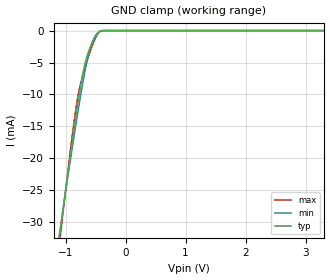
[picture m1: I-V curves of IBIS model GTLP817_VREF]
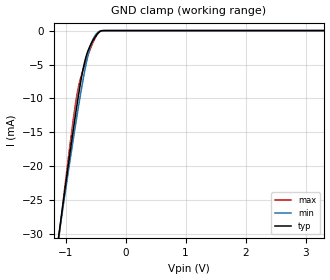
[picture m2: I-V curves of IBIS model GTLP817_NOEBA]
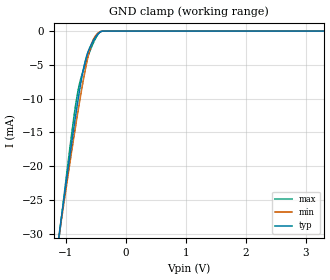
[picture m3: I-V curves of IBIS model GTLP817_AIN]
| TEXAS INSTRUMENTS INCORPORATED
| Standard Linear and Logic Group
| IBIS Model of SN74GTLP817
| GTLP-TO-LVTTL 1-TO-6 FANOUT DRIVER
| This file contains package information for the following:
|  TSSOP 24-pin (PW) package as [Component] GTLP817_PW
|  SOIC 24-pin (DW) package as [Component] GTLP817_DW
|  TVSOP 24-pin (DGV) package as [Component] GTLP817_DGV
| This device can be powered at the following Vccs:
|  3.3 volt Vcc
| This file provides unique models under the [Model Selector] for each Vcc.
| For operation at a specific Vcc, select the appropriate model after each
| [Model Selector] keyword.
[IBIS Ver]   3.2
[Comment char]  |_char
[File Name]   sn74gtlp817.ibs
[File Rev]   1.1 | c_die
[Date]   February 12, 2001
[Source]   Data created from TI-SPICE simulations at TI-SLL.
[Notes]   The following is an IBIS list for the GTLP817.
   Please contact sllibis@ti.com with questions and
   comments concerning SLL IBIS models.
   B_port output is simulated in Slow Mode(ERC=VCC)
   WARNING WHEN IBISCHK3.2.6 is Run
   -Pulldown Maximum data is non-monotonic
   -Pullup Maximum data is non-monotonic
   -Pullup Typical data is non-monotonic
   -Pullup Minimum data is non-monotonic
   -[Model] GTLP817_BOUT has no description of the
   buffer's high state DC drive characteristics
   (no [Pullup] table).This warning can be silenced
   by changing the Model_type or by adding a
   Pullup] table.
[Disclaimer] Property of Texas Instruments Incorporated.  Unauthorized
   reproduction and/or distribution is strictly prohibited.
   This product is protected under copyright law.
   Created  2001, (C) Copyright  2001, Texas Instruments
   Incorporated, All Rights Reserved
   UNLESS THERE IS A SIGNED, WRITTEN AGREEMENT TO THE
   CONTRARY, TEXAS INSTRUMENTS (TI) IS PROVIDING THE IBIS
   MODELS  AND WITHOUT ANY WARRANTY, EXPRESSED OR
   IMPLIED.  TI assumes no liability for:
   1) the accuracy of the IBIS models provided to your
   company;
   2) the proper functioning of these IBIS Models in your
   design or for any resulting applications; or
   3) infringement of patents, copyrights or intellectual
   property rights resulting from your use of these IBIS
   models.
   TI provides IBIS Models as a service to our customers.
   You and your company shall not distribute, sell or give
   these models to anyone else without prior written
   permission from TI.
   TI reserves the right to make changes to our products or
   to discontinue any semiconductor product or service
   without notice, and advises our customers to obtain the
   latest version of relevant information to verify, before
   placing orders, that the information being relied on is
   current.
   Please be aware that your receipt and use of the IBIS
   information provided shall serve as acceptance of these
   terms and conditions.  If you do not accept these terms,
   you should return or destroy the IBIS models and any
   other accompanying information immediately.
| Component GTLP817_PW 24-pin TSSOP
[Component]   GTLP817_PW
[Manufacturer]   Texas Instruments, Inc.
[Package]
|   typ   min   max
R_pkg   3.900e-02   3.000e-02   4.600e-02
L_pkg   2.685e-09   2.367e-09   3.177e-09
C_pkg   3.200e-13   2.520e-13   4.340e-13
[Pin]   signal_name   model_name   R_pin   L_pin   C_pin
1   AI   GTLP817_AIN   3.700e-02   3.153e-09   4.340e-13
2   AO1   GTLP817_AOUT   3.400e-02   2.629e-09   3.410e-13
3   GNDT   GND   3.200e-02   2.860e-09   3.470e-13
4   AO2   GTLP817_AOUT   4.200e-02   2.741e-09   2.900e-13
5   VCC   POWER   4.600e-02   2.600e-09   2.620e-13
6   AO3   GTLP817_AOUT   4.300e-02   2.414e-09   2.660e-13
7   GNDT   GND   4.200e-02   2.367e-09   2.620e-13
8   AO4   GTLP817_AOUT   4.400e-02   2.461e-09   2.520e-13
9   VCC   POWER   4.200e-02   2.543e-09   2.740e-13
10   AO5   GTLP817_AOUT   3.000e-02   2.616e-09   3.320e-13
11   GNDT   GND   3.700e-02   2.670e-09   3.460e-13
12   AO6   GTLP817_AOUT   3.900e-02   3.177e-09   4.330e-13
13   GNDT   GND   3.700e-02   3.111e-09   4.310e-13
14   NOEBA   GTLP817_NOEBA   3.700e-02   2.656e-09   3.450e-13
15   BI   GTLP817_BIN   3.100e-02   2.739e-09   3.400e-13
16   GNDG   GND   4.200e-02   2.649e-09   2.820e-13
17   BO2   GTLP817_BOUT   4.600e-02   2.532e-09   2.570e-13
18   ERC   GTLP817_ERC   4.400e-02   2.425e-09   2.660e-13
19   GNDG   GND   4.400e-02   2.425e-09   2.660e-13
20   VREF   GTLP817_VREF   4.600e-02   2.532e-09   2.570e-13
21   GNDG   GND   4.200e-02   2.648e-09   2.820e-13
22   BO1   GTLP817_BOUT   3.100e-02   2.738e-09   3.390e-13
23   NOEAB   GTLP817_NOEAB   3.600e-02   2.653e-09   3.440e-13
24   GNDT   GND   3.700e-02   3.110e-09   4.310e-13
| Component GTLP817_DW 24-pin SOIC
[Component]   GTLP817_DW
[Manufacturer]   Texas Instruments, Inc.
[Package]
|   typ   min   max
R_pkg   3.700e-02   3.000e-02   4.700e-02
L_pkg   5.146e-09   3.993e-09   6.885e-09
C_pkg   7.580e-13   5.120e-13   1.067e-12
[Pin]   signal_name   model_name   R_pin   L_pin   C_pin
1   AI   GTLP817_AIN   3.900e-02   6.885e-09   1.067e-12
2   AO1   GTLP817_AOUT   4.200e-02   5.950e-09   9.580e-13
3   GNDT   GND   4.700e-02   5.317e-09   7.910e-13
4   AO2   GTLP817_AOUT   3.100e-02   4.651e-09   6.110e-13
5   VCC   POWER   3.000e-02   3.993e-09   5.120e-13
6   AO3   GTLP817_AOUT   3.000e-02   4.083e-09   6.110e-13
7   GNDT   GND   3.000e-02   4.083e-09   6.110e-13
8   AO4   GTLP817_AOUT   3.000e-02   3.993e-09   5.120e-13
9   VCC   POWER   3.100e-02   4.652e-09   6.110e-13
10   AO5   GTLP817_AOUT   4.700e-02   5.317e-09   7.910e-13
11   GNDT   GND   4.200e-02   5.950e-09   9.590e-13
12   AO6   GTLP817_AOUT   3.900e-02   6.885e-09   1.067e-12
13   GNDT   GND   3.900e-02   6.885e-09   1.067e-12
14   NOEBA   GTLP817_NOEBA   4.200e-02   5.950e-09   9.590e-13
15   BI   GTLP817_BIN   4.700e-02   5.317e-09   7.910e-13
16   GNDG   GND   3.100e-02   4.652e-09   6.110e-13
17   BO2   GTLP817_BOUT   3.000e-02   3.993e-09   5.120e-13
18   ERC   GTLP817_ERC   3.000e-02   4.083e-09   6.100e-13
19   GNDG   GND   3.000e-02   4.083e-09   6.100e-13
20   VREF   GTLP817_VREF   3.000e-02   3.993e-09   5.120e-13
21   GNDG   GND   3.100e-02   4.651e-09   6.110e-13
22   BO1   GTLP817_BOUT   4.700e-02   5.317e-09   7.910e-13
23   NOEAB   GTLP817_NOEAB   4.200e-02   5.950e-09   9.580e-13
24   GNDT   GND   3.900e-02   6.885e-09   1.067e-12
| Component GTLP817_DGV 24-pin TVSOP
[Component]   GTLP817_DGV
[Manufacturer]   Texas Instruments, Inc.
[Package]
|   typ   min   max
R_pkg   4.300e-02   3.900e-02   4.700e-02
L_pkg   2.601e-09   2.312e-09   3.626e-09
C_pkg   3.580e-13   2.770e-13   5.950e-13
[Pin]   signal_name   model_name   R_pin   L_pin   C_pin
1   AI   GTLP817_AIN   4.300e-02   3.625e-09   5.950e-13
2   AO1   GTLP817_AOUT   4.000e-02   2.656e-09   4.020e-13
3   GNDT   GND   3.900e-02   2.338e-09   3.080e-13
4   AO2   GTLP817_AOUT   4.600e-02   2.354e-09   2.770e-13
5   VCC   POWER   4.500e-02   2.312e-09   2.850e-13
6   AO3   GTLP817_AOUT   4.700e-02   2.318e-09   2.820e-13
7   GNDT   GND   4.700e-02   2.318e-09   2.820e-13
8   AO4   GTLP817_AOUT   4.500e-02   2.312e-09   2.850e-13
9   VCC   POWER   4.600e-02   2.353e-09   2.780e-13
10   AO5   GTLP817_AOUT   3.900e-02   2.338e-09   3.080e-13
11   GNDT   GND   4.100e-02   2.660e-09   4.020e-13
12   AO6   GTLP817_AOUT   4.300e-02   3.625e-09   5.950e-13
13   GNDT   GND   4.400e-02   3.626e-09   5.940e-13
14   NOEBA   GTLP817_NOEBA   4.000e-02   2.658e-09   4.020e-13
15   BI   GTLP817_BIN   3.900e-02   2.343e-09   3.110e-13
16   GNDG   GND   4.600e-02   2.353e-09   2.780e-13
17   BO2   GTLP817_BOUT   4.500e-02   2.312e-09   2.850e-13
18   ERC   GTLP817_ERC   4.700e-02   2.319e-09   2.820e-13
19   GNDG   GND   4.700e-02   2.319e-09   2.820e-13
20   VREF   GTLP817_VREF   4.500e-02   2.312e-09   2.850e-13
21   GNDG   GND   4.600e-02   2.353e-09   2.780e-13
22   BO1   GTLP817_BOUT   3.900e-02   2.337e-09   3.080e-13
23   NOEAB   GTLP817_NOEAB   4.000e-02   2.658e-09   4.020e-13
24   GNDT   GND   4.400e-02   3.626e-09   5.950e-13
| Models and submodels in the file (8): GTLP817_VREF (Input), GTLP817_NOEBA (Input), GTLP817_AIN (Input), GTLP817_NOEAB (Input), GTLP817_BIN (Input), GTLP817_ERC (Input), GTLP817_AOUT (3-state), GTLP817_BOUT (Open_drain)
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| NOTE:  The [Diff Pin] section is commented out because the ibischk3 program
|   currently flags it as an Error when it shouldn't
| [Diff Pin]  inv_pin   vdiff   tdelay_typ
|15   20   100mv   NA
|22   20   100mv   NA
|17   20   100mv   NA
[Model]   GTLP817_VREF
Model_type  Input
Vinl=0.8
Vinh=2.0
| variable   typ   min   max
C_comp   4.55pF   3.67pF   5.26pF
[Temperature Range]   40   100   -40
| Ambient temperature   25   85   -40
[Voltage range]   3.3   3.15   3.45
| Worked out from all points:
|   GND clamp passes 1 mA (typ) near -0.50 V on its own axis
[GND Clamp]
| GTLP817_VREF
|   Voltage   I(typ)   I(min)   I(max)
-5.5V     -377.3mA   -344.1mA   -427.7mA
-1.09V    -31.42mA   -31.13mA   -32.42mA
-1.05V    -28.57mA   -28.54mA   -29.16mA
-865mV    -15.86mA   -16.94mA   -14.73mA
-825mV    -13.28mA   -14.55mA   -12.05mA
-785mV    -10.81mA   -12.22mA   -9.84mA
-730mV    -7.69mA    -9.145mA   -7.617mA
-685mV    -5.554mA   -6.804mA   -6.095mA
-600mV    -2.893mA   -3.123mA   -3.532mA
-525mV    -1.39mA    -1.163mA   -1.661mA
-430mV    -167.4uA   -111.4uA   -160.9uA
3.3V      270.1pA    967.8pA    1.797nA
[Model]   GTLP817_NOEBA
Model_type  Input
Vinl=0.8
Vinh=2.0
| variable   typ   min   max
C_comp   2.71pF   2.00pF   3.85pF
[Temperature Range]   40   100   -40
| Ambient temperature   25   85   -40
[Voltage range]   3.3   3.15   3.45
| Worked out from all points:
|   GND clamp passes 1 mA (typ) near -0.51 V on its own axis
[GND Clamp]
| GTLP817_NOEBA
|   Voltage   I(typ)   I(min)   I(max)
-5.5V     -349.9mA   -322.6mA   -391.6mA
-1.135V   -31.72mA   -31.74mA   -32.32mA
-1.095V   -29.05mA   -29.29mA   -29.29mA
-900mV    -16.41mA   -17.67mA   -15.06mA
-835mV    -12.45mA   -13.97mA   -10.86mA
-790mV    -9.847mA   -11.49mA   -8.536mA
-690mV    -4.948mA   -6.385mA   -5.276mA
-605mV    -2.528mA   -2.9mA     -3.115mA
-540mV    -1.394mA   -1.229mA   -1.719mA
-450mV    -300.1uA   -191.4uA   -334.8uA
-360mV    -3.423uA   -9.411uA   -3.546uA
3.3V      169.1pA    605.3pA    1.317nA
[Model]   GTLP817_AIN
Model_type  Input
Vinl=0.8
Vinh=2.0
| variable   typ   min   max
C_comp   2.86pF   2.09pF   4.05pF
[Temperature Range]   40   100   -40
| Ambient temperature   25   85   -40
[Voltage range]   3.3   3.15   3.45
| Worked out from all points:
|   GND clamp passes 1 mA (typ) near -0.51 V on its own axis
[GND Clamp]
| GTLP817_AIN
|   Voltage   I(typ)   I(min)   I(max)
-5.5V     -349.9mA   -322.6mA   -391.6mA
-1.135V   -31.72mA   -31.74mA   -32.32mA
-1.095V   -29.05mA   -29.29mA   -29.29mA
-900mV    -16.41mA   -17.67mA   -15.06mA
-835mV    -12.45mA   -13.97mA   -10.86mA
-790mV    -9.847mA   -11.49mA   -8.536mA
-690mV    -4.948mA   -6.385mA   -5.276mA
-605mV    -2.528mA   -2.9mA     -3.115mA
-540mV    -1.394mA   -1.229mA   -1.719mA
-450mV    -300.1uA   -191.4uA   -334.8uA
-360mV    -3.423uA   -9.411uA   -3.546uA
3.3V      169.1pA    605.3pA    1.317nA
